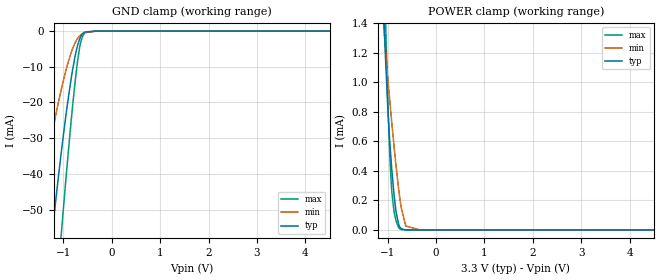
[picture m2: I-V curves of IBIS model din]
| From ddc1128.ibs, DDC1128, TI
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|   din Model
[Model]   din
Model_type   Input
Vinl = 0.66
Vinh = 2.64
|   typ   min   max
|   (nom PVT)   (fast PVT)   (slow PVT)
C_comp   1.650e-12   1.346e-12   1.978e-12
[Model spec]
|Subparameter
Vinl   0.66   0.54   0.72
Vinh   2.64   2.16   2.88
| Where nom  PVT is Nominal Process, 3.3V, 27C
|   Fast PVT is Strong Process,  3.6V, -40C
|   Slow PVT is Weak Process,   2.7V, 125C
[Voltage Range]   3.3   2.7   3.6
|Junction Temperature
[Temperature Range]   27   125   -40
[Power Clamp Reference]   3.3   2.7   3.6
[GND Clamp Reference]   0   0   0
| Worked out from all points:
|   GND clamp passes 1 mA (typ) near -0.62 V on its own axis
|   POWER clamp passes 1 mA (typ) near -1.02 V on its own axis
[GND Clamp]
|   Voltage   I(typ)   I(min)   I(max)
-3.3V     -364.2mA   -235.6mA   -458.5mA
-1.777V   -131.9mA   -73.56mA   -185.5mA
-1.482V   -89.65mA   -47.61mA   -132.5mA
-1.251V   -58.75mA   -29.79mA   -91.71mA
-1.165V   -47.99mA   -23.85mA   -76.87mA
-1.033V   -32.49mA   -15.57mA   -54.71mA
-929.4mV  -21.5mA    -9.962mA   -38.22mA
-837.6mV  -12.95mA   -5.873mA   -24.6mA
-732.6mV  -5.318mA   -2.586mA   -10.93mA
-643.2mV  -1.528mA   -1.06mA    -3.103mA
-556.8mV  -248.4uA   -384uA     -424.6uA
6.6V      0A         0A         0A
[POWER Clamp]
|   Voltage   I(typ)   I(min)   I(max)
-3.3V     30.39mA    23.73mA    37.34mA
-1.069V   1.367mA    1.325mA    1.734mA
-1.046V   1.174mA    1.225mA    1.441mA
-999.6mV  837.1uA    1.036mA    898.8uA
-956.4mV  595.2uA    873.3uA    505.7uA
-910.8mV  391.3uA    710.3uA    246.3uA
-826.8mV  122.1uA    432.2uA    59.96uA
-772.8mV  37.2uA     275.5uA    15.35uA
-719.4mV  8.213uA    148.7uA    2.577uA
-627mV    489.9nA    26.81uA    119.3nA
-330mV    0A         0A         0A
6.6V      0A         0A         0A
